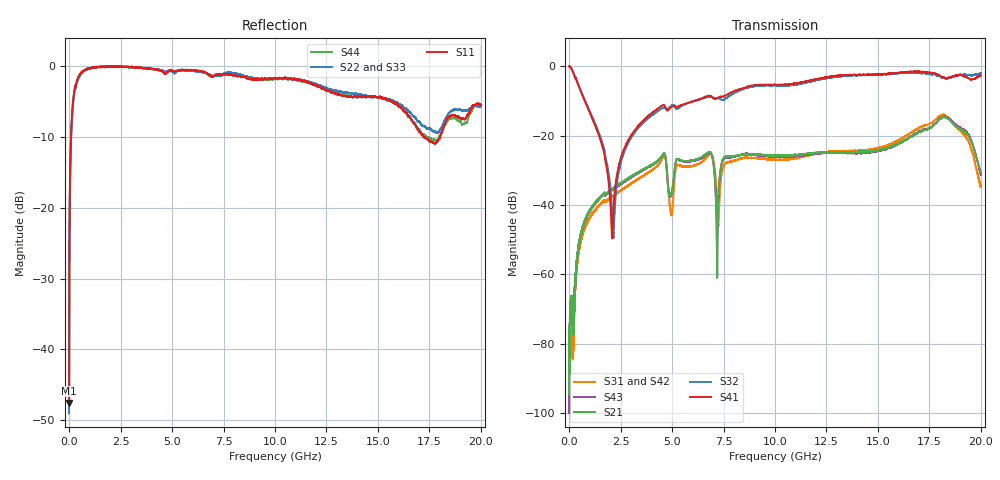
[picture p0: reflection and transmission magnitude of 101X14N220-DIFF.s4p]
!{101X14N220}
!Johanson Technology Inc.
!www.johansontechnology.com
!Test Board Conditions:
!Substrate Type  RO4350B
!Substrate Thickness  10 mil
!Substrate Dk  3.66
!TL Type: GCPW
!TL Trace Width  20 mil
!TL Gap  15 mil
!PART MODE DIFFERENTIAL
!DUT TOPOLOGY	DIFFERENTIAL 4-PORT
!Mounting Pad LxW  20x35 mil
# MHz S  dB  R 50
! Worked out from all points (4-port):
!   20001 points, 300 kHz to 20 GHz, reference 50 ohm
!   strongest paths, dB at 300 kHz, 5 GHz, 10 GHz, 15 GHz, 20 GHz:
!     S41: 0.0, -11.7, -5.3, -2.4, -2.7
!     S32: -0.1, -11.3, -5.6, -2.5, -2.0
!     S21: -82.2, -35.9, -25.7, -24.3, -30.8
!     S43: -87.9, -36.2, -26.1, -24.5, -31.3
!     S31: -80.4, -42.5, -26.9, -23.7, -34.8
!     S42: -84.9, -42.2, -26.8, -23.7, -34.8
!   lowest |S11| = -47.6 dB at 300 kHz (marker M1), VSWR 1.01, Z = 50.1 - j0.401 ohm
!   |S11| at or under -10 dB: start of sweep to 93.31 MHz; 17.23009 GHz to 17.233 GHz (2.91 MHz wide, 0.0169 % of centre); 17.23 GHz to 18.02 GHz (789.1 MHz wide, 4.48 % of centre)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
0.3  -47.60 -73.7  -86.81 85.6  -81.61 -29.0  -0.05 0.2
     -82.17 -165.2  -49.06 -62.6  -0.04 0.0  -82.59 63.2
     -80.41 -8.1  -0.07 0.2  -45.39 -62.9  -86.11 -120.6
     -0.04 0.2  -84.86 96.3  -87.89 68.7  -47.39 -67.2
288.296  -2.85 -138.9  -63.58 143.2  -63.58 -169.6  -3.30 -48.6
         -64.00 153.2  -3.08 -138.1  -3.19 -47.6  -65.57 -174.6
         -63.60 -178.3  -3.20 -47.7  -2.93 -138.1  -62.25 143.1
         -3.31 -48.6  -62.30 -167.0  -63.86 145.4  -2.84 -139.2
2150.268  -0.03 168.5  -35.15 78.3  -37.27 77.5  -41.83 54.7
          -35.20 78.2  -0.03 171.7  -49.20 -4.9  -37.40 79.0
          -37.33 77.5  -49.35 -6.1  -0.01 170.7  -35.47 78.9
          -41.80 54.8  -37.35 78.9  -35.49 78.7  -0.05 170.3
4543.232  -0.75 147.3  -25.55 30.4  -26.46 23.1  -11.25 50.0
          -25.54 30.5  -0.59 148.4  -12.08 53.0  -26.79 22.7
          -26.42 23.3  -12.04 53.1  -0.52 146.6  -25.70 28.4
          -11.25 49.8  -26.79 22.3  -25.70 28.0  -0.74 145.3
7197.192  -1.14 133.8  -52.20 71.9  -40.35 -125.5  -9.18 29.1
          -52.57 69.3  -1.32 123.7  -9.20 21.8  -40.77 -130.1
          -40.36 -124.6  -9.18 22.0  -1.27 123.9  -56.36 127.4
          -9.22 28.9  -40.76 -130.4  -56.03 127.0  -1.14 124.0
18209.03  -8.43 65.4  -14.64 148.6  -14.07 148.3  -3.32 -62.4
          -14.68 148.3  -7.85 75.1  -3.45 -55.3  -13.71 153.3
          -13.99 148.8  -3.39 -54.5  -6.99 70.0  -14.49 146.0
          -3.28 -62.1  -13.70 153.9  -14.52 145.8  -8.44 68.9
20000  -5.49 45.3  -30.81 -38.2  -34.88 -81.8  -2.71 -58.8
       -30.80 -37.9  -5.72 46.7  -2.08 -55.1  -34.83 -82.0
       -34.76 -81.5  -2.02 -54.4  -5.86 37.3  -31.29 -42.1
       -2.69 -58.5  -34.77 -82.3  -31.31 -42.2  -5.39 40.5
